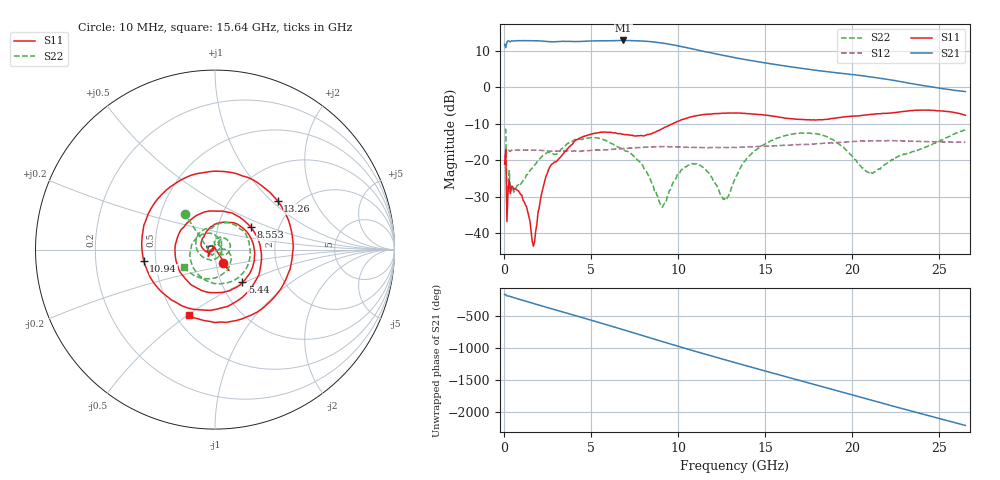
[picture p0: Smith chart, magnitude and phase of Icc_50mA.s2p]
!Keysight Technologies,N5245A,MY52451697,A.10.60.06
!Date: Thursday, May 06, 2021 15:04:21
!Correction: S11(Full 2 Port(1,4))
!S41(Full 2 Port(1,4))
!S14(Full 2 Port(1,4))
!S44(Full 2 Port(1,4))
!S2P File: Measurements: S11, S41, S14, S44:
# Hz S  dB  R 50
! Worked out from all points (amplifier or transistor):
!   401 points, 10 MHz to 26.5 GHz, reference 50 ohm
!   highest |S21| = 12.8 dB at 6.831 GHz (marker M1)
!   |S21| within 3 dB of that: start of sweep to 11.47 GHz
!   unconditionally stable (mu >= 1): start of sweep to end of sweep
!   at 4.381 GHz: K = 1.13, MAG = 12.8 dB, |S12| = -17.5 dB
!   at 13.26 GHz: K = 1.23, MAG = 9.4 dB, |S12| = -16.5 dB
!   at 26.5 GHz: K = 2.52, MAG = 0.1 dB, |S12| = -15.1 dB
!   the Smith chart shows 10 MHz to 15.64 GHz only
!   S11 on the Smith chart (normalised r, x): 10 MHz: 1.08, -0.16; 5.44 GHz: 1.26, -0.48; 8.553 GHz: 1.44, +0.38; 10.94 GHz: 0.43, -0.06; 13.26 GHz: 1.62, +1.09; 15.64 GHz: 0.58, -0.51
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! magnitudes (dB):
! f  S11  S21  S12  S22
! 10 MHz  -21.1  11.7  -18.8  -11.7
! 274.9 MHz  -25.4  12.5  -17.4  -22.9
! 473.6 MHz  -27.2  12.6  -17.3  -27.6
! 1.136 GHz  -31.4  12.7  -17.2  -25.3
! 1.666 GHz  -43.5  12.7  -17.2  -21.8
! 2.527 GHz  -22.7  12.4  -17.5  -17.9
! 4.447 GHz  -13.7  12.5  -17.5  -14.3
! 5.44 GHz  -12.5  12.7  -17.2  -14.0
! 6.831 GHz  -12.9  12.8  -16.8  -17.2
! 8.553 GHz  -12.5  12.3  -16.4  -27.0
! 8.884 GHz  -11.9  12.2  -16.3  -31.1
! 9.149 GHz  -11.2  12.0  -16.3  -32.2
! 10.08 GHz  -9.2  11.2  -16.4  -23.5
! 10.94 GHz  -7.9  10.3  -16.5  -21.0
! 12.66 GHz  -7.1  8.6  -16.5  -30.5
! 13.26 GHz  -7.1  8.0  -16.5  -25.1
! 14.25 GHz  -7.4  7.2  -16.3  -18.0
! 15.64 GHz  -8.1  6.1  -16.1  -14.0
! 17.69 GHz  -9.0  4.7  -15.6  -12.7
! 20.87 GHz  -7.6  2.9  -14.7  -23.2
! 22.13 GHz  -7.1  2.0  -14.7  -20.3
! 26.5 GHz  -7.7  -1.2  -15.1  -11.7
